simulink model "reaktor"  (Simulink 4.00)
settings: Solver=ode45  StartTime=0.0  StopTime=50000  FixedStep=Ts  RelTol=1e-3
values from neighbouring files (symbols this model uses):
  c_p = 4200    [sim_reaktor.m]
  lambda = 420    [sim_reaktor.m]
  lambda_0 = 84    [sim_reaktor.m]
  m = 600    [sim_reaktor.m]
  m_p = 40    [sim_reaktor.m]
  Phi_p = 1.6    [sim_reaktor.m]
  S = 2    [sim_reaktor.m]
  T_0 = 17    [sim_reaktor.m]
  T_h = 12    [sim_reaktor.m]
  T_v = 75    [sim_reaktor.m]
  Theta_Pzac = 10    [sim_reaktor.m]
  Theta_zac = 10    [sim_reaktor.m]
  var_noise = 0.00001    (= 1e-05)    [sim_reaktor.m]

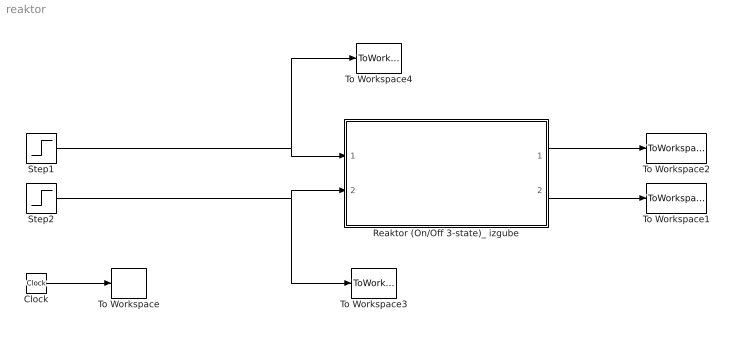
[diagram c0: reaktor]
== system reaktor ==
  Clock : Clock
  Reaktor (On/Off 3-state)_ izgube : Subsystem
  Step1 : Step  Time=5000  Before=-1  After=1  SampleTime=0
  Step2 : Step  Time=5000  Before=0  After=0.1  SampleTime=0
  To Workspace : ToWorkspace  VariableName=t  SampleTime=-1  SaveFormat=Array
  To Workspace1 : ToWorkspace  VariableName=mv2  SampleTime=-1  SaveFormat=Array
  To Workspace2 : ToWorkspace  VariableName=mv1  SampleTime=-1  SaveFormat=Array
  To Workspace3 : ToWorkspace  VariableName=cv2  SampleTime=-1  SaveFormat=Array
  To Workspace4 : ToWorkspace  VariableName=cv1  SampleTime=-1  SaveFormat=Array
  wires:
  Clock/1 -> To Workspace/1
  Reaktor (On/Off 3-state)_ izgube/1(Theta) -> To Workspace2/1
  Reaktor (On/Off 3-state)_ izgube/2(Theta_Pizh) -> To Workspace1/1
  Step1/1 -> Reaktor (On/Off 3-state)_ izgube/1(On/Off Ventil / hladna=0; vroca=1), To Workspace4/1
  Step2/1 -> Reaktor (On/Off 3-state)_ izgube/2(Servo ventil 0-1), To Workspace3/1

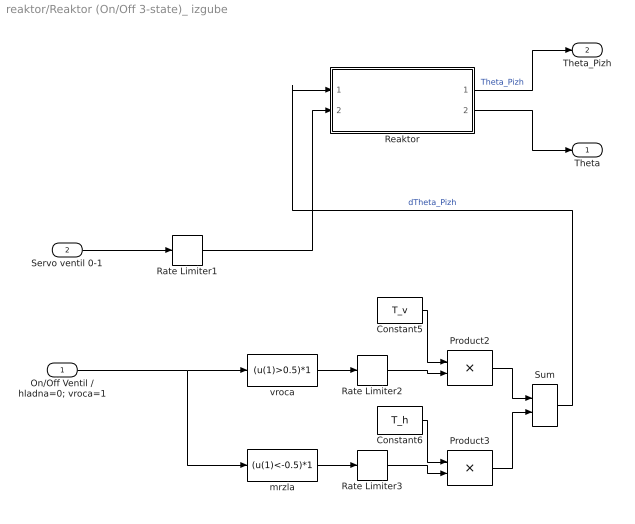
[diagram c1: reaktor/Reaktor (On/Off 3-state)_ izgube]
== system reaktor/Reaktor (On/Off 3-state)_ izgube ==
  On/Off Ventil / hladna=0; vroca=1 : Inport  Port=1  LatchInput=off
  Servo ventil 0-1 : Inport  Port=2  LatchInput=off
  Constant5 : Constant  Value=T_v
  Constant6 : Constant  Value=T_h
  Product2 : Product  Inputs=2  Multiplication=Element-wise(.*)  SaturateOnIntegerOverflow=on
  Product3 : Product  Inputs=2  Multiplication=Element-wise(.*)  SaturateOnIntegerOverflow=on
  Rate Limiter1 : RateLimiter  RisingSlewLimit=1/100  FallingSlewLimit=-1/100
  Rate Limiter2 : RateLimiter  RisingSlewLimit=1/60  FallingSlewLimit=-1/60
  Rate Limiter3 : RateLimiter  RisingSlewLimit=.016  FallingSlewLimit=-.016
  Reaktor : Subsystem
  Sum : Sum  Inputs=++  SaturateOnIntegerOverflow=on
  mrzla : Fcn  Expr=(u(1)<-0.5)*1
  vroca : Fcn  Expr=(u(1)>0.5)*1
  Theta : Outport  Port=1
  Theta_Pizh : Outport  Port=2
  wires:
  Reaktor/1(Theta_Pizh) -> Theta_Pizh/1  "Theta_Pizh"
  Reaktor/2(Theta) -> Theta/1
  Servo ventil 0-1/1 -> Rate Limiter1/1
  vroca/1 -> Rate Limiter2/1
  mrzla/1 -> Rate Limiter3/1
  Rate Limiter2/1 -> Product2/2
  Rate Limiter3/1 -> Product3/2
  Constant5/1 -> Product2/1
  Constant6/1 -> Product3/1
  Product2/1 -> Sum/1
  Product3/1 -> Sum/2
  Sum/1 -> Reaktor/1(Theta_Pvh)  "dTheta_Pizh"
  On/Off Ventil / hladna=0; vroca=1/1 -> vroca/1, mrzla/1
  Rate Limiter1/1 -> Reaktor/2(Ventil)

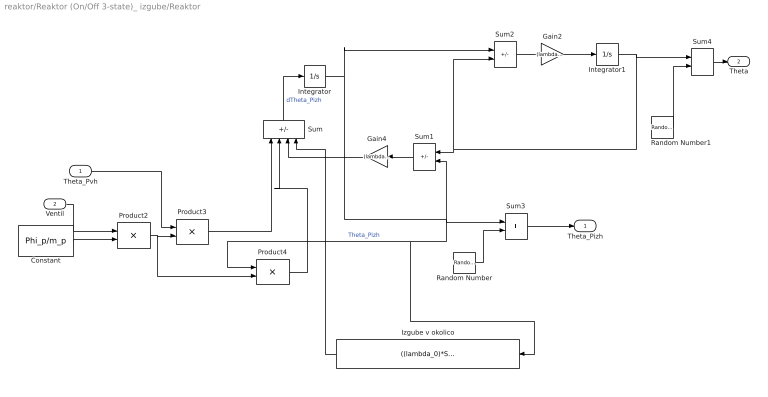
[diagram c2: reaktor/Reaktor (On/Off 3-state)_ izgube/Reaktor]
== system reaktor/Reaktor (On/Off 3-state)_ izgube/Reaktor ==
  Theta_Pvh : Inport  Port=1  LatchInput=off
  Ventil : Inport  Port=2  LatchInput=off
  Constant : Constant  Value=Phi_p/m_p
  Gain2 : Gain  Gain=(lambda*S)/(m*c_p)  Multiplication=Element-wise(K.*u)  SaturateOnIntegerOverflow=on
  Gain4 : Gain  Orientation=left  Gain=(lambda*S)/(m_p*c_p)  Multiplication=Element-wise(K.*u)  SaturateOnIntegerOverflow=on
  Integrator : Integrator  ExternalReset=none  InitialConditionSource=internal  InitialCondition=Theta_Pzac  LimitOutput=off  UpperSaturationLimit=inf  LowerSaturationLimit=-inf  ShowSaturationPort=off  ShowStatePort=off  AbsoluteTolerance=auto
  Integrator1 : Integrator  ExternalReset=none  InitialConditionSource=internal  InitialCondition=Theta_zac  LimitOutput=off  UpperSaturationLimit=inf  LowerSaturationLimit=-inf  ShowSaturationPort=off  ShowStatePort=off  AbsoluteTolerance=auto
  Izgube v okolico : Fcn  Orientation=left  Expr=((lambda_0)*S)/(m_p*c_p)*(u(1)-T_0)
  Product2 : Product  Inputs=2  Multiplication=Element-wise(.*)  SaturateOnIntegerOverflow=on
  Product3 : Product  Inputs=2  Multiplication=Element-wise(.*)  SaturateOnIntegerOverflow=on
  Product4 : Product  Inputs=2  Multiplication=Element-wise(.*)  SaturateOnIntegerOverflow=on
  Random Number : RandomNumber  Mean=0  Variance=var_noise  Seed=0  SampleTime=0
  Random Number1 : RandomNumber  Mean=0  Variance=var_noise  Seed=1  SampleTime=0
  Sum : Sum  Orientation=up  Inputs=+---  SaturateOnIntegerOverflow=on
  Sum1 : Sum  Orientation=left  Inputs=-+  SaturateOnIntegerOverflow=on
  Sum2 : Sum  Inputs=+-  SaturateOnIntegerOverflow=on
  Sum3 : Sum  Inputs=++  SaturateOnIntegerOverflow=on
  Sum4 : Sum  Inputs=++  SaturateOnIntegerOverflow=on
  Theta_Pizh : Outport  Port=1
  Theta : Outport  Port=2
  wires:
  Constant/1 -> Product2/2
  Ventil/1 -> Product2/1
  Product2/1 -> Product3/2, Product4/2
  Theta_Pvh/1 -> Product3/1
  Product3/1 -> Sum/1
  Product4/1 -> Sum/2
  Sum1/1 -> Gain4/1
  Gain4/1 -> Sum/3
  Sum/1 -> Integrator/1  "dTheta_Pizh"
  Integrator/1 -> Sum1/2, Sum3/1, Product4/1, Izgube v okolico/1, Sum2/1  "Theta_Pizh"
  Sum2/1 -> Gain2/1
  Gain2/1 -> Integrator1/1
  Integrator1/1 -> Sum1/1, Sum2/2, Sum4/1
  Sum3/1 -> Theta_Pizh/1
  Sum4/1 -> Theta/1
  Random Number/1 -> Sum3/2
  Random Number1/1 -> Sum4/2
  Izgube v okolico/1 -> Sum/4
